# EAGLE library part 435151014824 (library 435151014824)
Tactile Switches WS-TASV Tact Switch Source: Datasheet
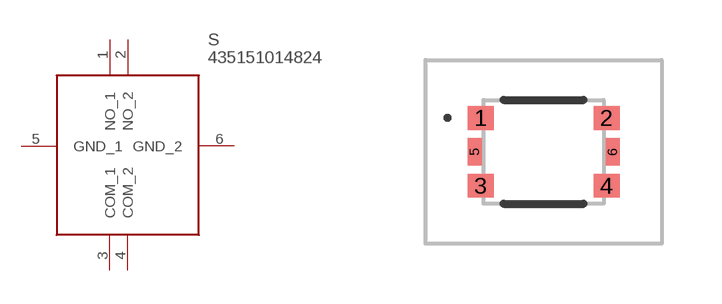
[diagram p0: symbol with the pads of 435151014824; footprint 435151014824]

Designator prefix S

## 435151014824 (Description: Tactile Switches WS-TASV Tact Switch; Height: 1.4mm; Manufacturer_Name: Wurth Elektronik; Manufacturer_Part_Number: 435151014824; Mouser_Part_Number: 710-435151014824; Mouser_Price-Stock: https://www.mouser.co.uk/ProductDetail/Wurth-Elektronik/435151014824?qs=OlC7AqGiEDkCCtReGm3ZVw%3D%3D)  [435151014824]
1  NO_1
2  NO_2
3  COM_1
4  COM_2
5  GND_1
6  GND_2

## Footprint 435151014824 (pad centres in mm)
435151014824-2
smd 0.65 x 0.6: 1 -1.575,0.85; 2 1.575,0.85; 3 -1.575,-0.85; 4 1.575,-0.85
smd 0.35 x 0.7: 5 -1.725,0; 6 1.725,0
